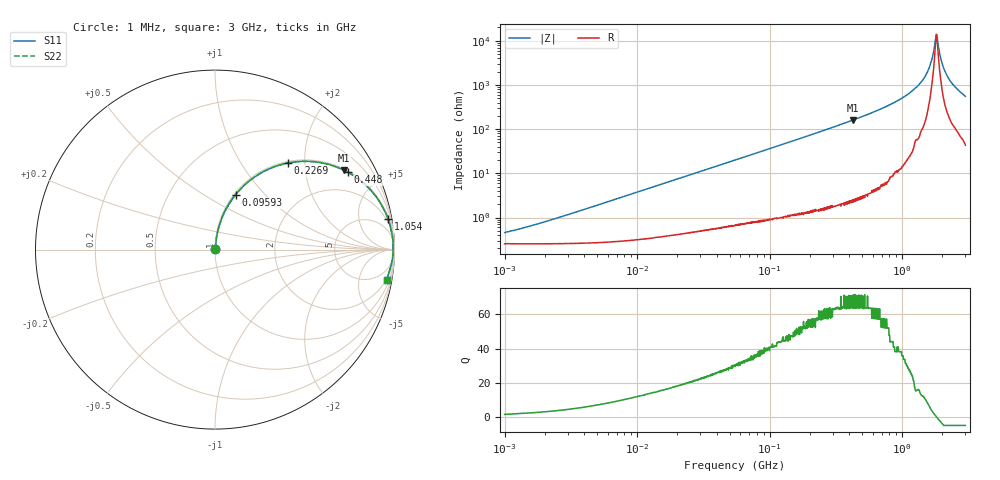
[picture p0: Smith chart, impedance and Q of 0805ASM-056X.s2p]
!s-Parameter Generated by FASTRON Sdn. Bhd.
!FASTRON P/N : 0805ASM-056X
!Keysight Technologies: E4991B_MY54100416_A.01.15
!Date: Fri Jun 19 14:49:14 2026
!Version  :Rev00  Fri Jun 19 14:49:14 2026
!Data & Calibration Information:
!Freq  S11  S21  S12  S22
!PortZ  Port1:50+j0  Port2:50+j0
!When reading reference impedance value at option line is always used.
! Remarks : This data is being provided solely for informational purposes.
# Hz S dB R 50
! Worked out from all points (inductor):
!   1601 points, 1 MHz to 3 GHz, reference 50 ohm
!   read as one part in series: L = 60.3 nH near 2.025 MHz
!   highest Q = 70.7 at 428.3 MHz (marker M1), where L = 60.1 nH
!   self-resonance near 1.81 GHz
!   S11 on the Smith chart (normalised r, x): 1 MHz: 1.01, +0.01; 95.93 MHz: 1.02, +0.70; 226.9 MHz: 1.03, +1.65; 448 MHz: 1.06, +3.40; 1.054 GHz: 1, +11; 3 GHz: 2, -11
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1000000  -46.80 56.0  -0.02 -0.2  -0.02 -0.2  -46.80 56.0
3804036  -36.70 78.8  -0.02 -0.8  -0.02 -0.8  -36.70 78.8
1.447069e7  -25.40 83.1  -0.04 -3.1  -0.04 -3.1  -25.40 83.1
5.504702e7  -14.20 76.8  -0.23 -11.3  -0.23 -11.3  -14.20 76.8
9.593103e7  -9.73 69.5  -0.56 -19.0  -0.56 -19.0  -9.73 69.5
2.083556e8  -4.46 52.2  -2.04 -36.8  -2.04 -36.8  -4.46 52.2
2.268557e8  -3.99 49.8  -2.33 -39.2  -2.33 -39.2  -3.99 49.8
4.282981e8  -1.46 31.5  -5.64 -57.7  -5.64 -57.7  -1.46 31.5
4.480278e8  -1.35 30.2  -5.96 -58.9  -5.96 -58.9  -1.35 30.2
7.925923e8  -0.39 16.0  -11.20 -72.9  -11.20 -72.9  -0.39 16.0
1.054198e9  -0.18 10.1  -15.10 -78.1  -15.10 -78.1  -0.18 10.1
1.307284e9  -0.11 6.0  -19.60 -80.4  -19.60 -80.4  -0.11 6.0
1.488926e9  -0.07 3.6  -23.90 -81.0  -23.90 -81.0  -0.07 3.6
1.629261e9  -0.06 1.9  -29.20 -77.1  -29.20 -77.1  -0.06 1.9
1.687342e9  -0.06 1.3  -32.30 -71.5  -32.30 -71.5  -0.06 1.3
1.76507e9  -0.06 0.5  -38.70 -52.0  -38.70 -52.0  -0.06 0.5
1.818868e9  -0.06 -0.0  -42.90 5.5  -42.90 5.5  -0.06 -0.0
1.86495e9  -0.07 -0.5  -38.70 48.5  -38.70 48.5  -0.07 -0.5
2.01032e9  -0.08 -1.9  -29.40 74.3  -29.40 74.3  -0.08 -1.9
2.188818e9  -0.10 -3.5  -24.10 77.9  -24.10 77.9  -0.10 -3.5
2.492946e9  -0.16 -6.1  -19.40 77.2  -19.40 77.2  -0.16 -6.1
3e9  -0.26 -10.1  -15.10 75.4  -15.10 75.4  -0.26 -10.1
